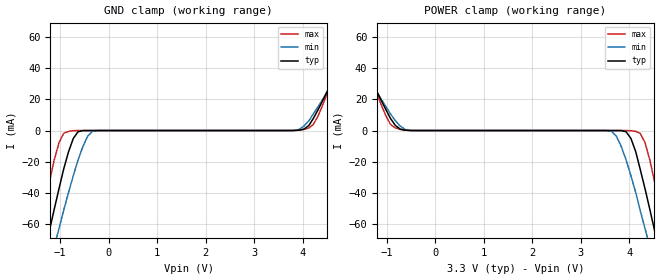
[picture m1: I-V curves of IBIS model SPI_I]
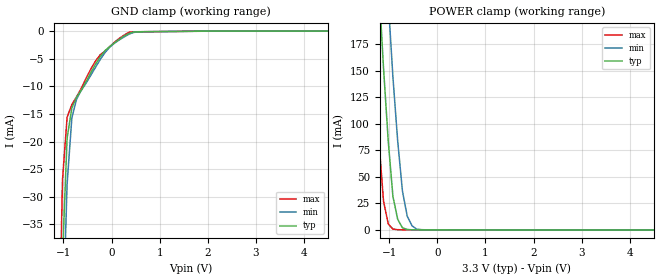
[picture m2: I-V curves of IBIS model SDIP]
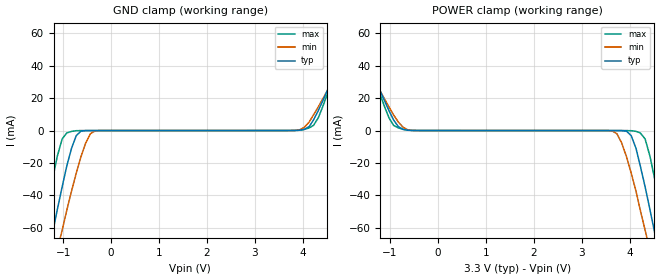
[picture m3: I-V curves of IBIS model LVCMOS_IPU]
|   National Semiconductor Corporation
|   IBIS Model of LMH0387
[IBIS Ver]   4.2
[File name]   lmh0387.ibs
[File Rev]   1.2
[Notes]
 Created By  Pegah Alavi
   Revision History
   1.0  Initial Release
   1.1  Updated SDOP/SDON buffer
   1.2  Updated SPDP and SPIN C_comp values
This model supports the LVCMOS output, LVCMOS Input, SPI input, SPI
output, CML input, and LVDS output on the LMH0387. Static, analog,
and reserved pins are not modeled. Note that the SDIP and SDIN pins
need an external 100ohm termination.
Begin IBIS Parser Results
| Do NOT edit this section manually!
Checking ...\LMH0387.ibs for IBIS 4.2 Compatibility...
WARNING - Combined Pulldown for Model: SDON Typical data is non-monotonic
WARNING - Combined Pulldown for Model: SDON Minimum data is non-monotonic
WARNING - Combined Pulldown for Model: SDON Maximum data is non-monotonic
WARNING - Combined Pulldown for Model: SDOP Typical data is non-monotonic
WARNING - Combined Pulldown for Model: SDOP Minimum data is non-monotonic
WARNING - Combined Pulldown for Model: SDOP Maximum data is non-monotonic
Errors  : 0
Warnings: 6
File Passed
| End IBIS Parser Results
[Date]   09/15/2010
[Source]  Generated by National Semincoductor Corporation.
[Disclaimer]
(C) Copyright National Semiconductor Corporation 2010
   All rights reserved
National Semiconductor Corporation hereby grants the
user of this IBIS model a non-exclusive, nontransferable
license to use this IBIS model under the following terms.
Before using this IBIS model, the user should read this
license.  If the user does not accept these terms,  the
IBIS model should be returned to National within 30 days.
The user is granted this license only to use the
IBIS model and is not granted rights to sell, load, rent,
lease or license the IBIS model in whole or in part, or in
modified form to anyone other than user. User may modify
the IBIS model to suit its specific applications but rights
to derivative works and such modifications shall belong to
National.
This IBIS model is provided on an "AS IS" basis and
National makes absolutely no warranty with respect to the
information contained herein.NATIONAL DISCLAIMS AND CUSTOMER
WAIVES ALL WARRANTIES, EXPRESS OR IMPLIED, INCLUDING
WARRANTIES OF MERCHANTABILITY OR FITNESS FOR A PARTICULAR
PURPOSE. The entire risk as to quality and performance is
with the Customer. ACCORDINGLY, IN NO EVENT SHALL THE
COMPANY BE LIABLE FOR ANY DAMAGES, WHETHER IN CONTRACT OR
TORT,INCLUDING ANY LOST PROFITS OR OTHER INCIDENTAL,
CONSEQUENTIAL, EXEMPLARY, OR PUNITIVE DAMAGES ARISING OUT
OF THE USE OR APPLICATION OF THE IBIS model provided in
this package.Further, National reserves the right to make
changes without notice to any product herein to improve
reliability, function, or design. National does not convey
any license under patent rights or any other intellectual
property rights, including those of third parties.
National is not obligated to provide maintenance or support
for the licensed IBIS model.
[Copyright]  Copyright 2010, National Semiconductor, All Rights Reserved
[Component]  LMH0387
[Manufacturer]  National Semiconductor Corp
[Package]
|   typ   min   max
R_pkg   0   0   0
L_pkg   0   0   0
C_pkg   0   0   0
[Pin]   signal_name   model_name   R_pin   L_pin   C_pin
1   RSVD   NC
2   VCCTX   POWER   1.80e-2   2.969e-10   6.261e-13
3   VCCTX   POWER   1.80e-2   2.969e-10   6.261e-13
4   RSVD   NC
5   RSVD   NC
6   RSVD   NC
7   RSVD   NC
8   BNC_IO   NC   1.60e-2   1.855e-10   3.405e-13
9   RSVD   NC
10   RSVD   NC
11   RSVD   NC
12   RSVD   NC
13   RSVD   NC
14   RSVD   NC
15   RSVD   NC
16   RSVD   NC
17   TERMRX   NC   2.77e-1   1.679e-09   2.691e-13
18   SPI_EN   NC   2.87e-1   1.486e-09   1.329e-13
19   VEE   GND   3.00e-2   2.116e-10   3.185e-12
20   AECP   NC   2.93e-1   1.179e-09   1.128e-13
21   AECN   NC   2.76e-1   1.062e-09   1.103e-13
22   CDB   LVCMOS_O   2.66e-1   1.020e-09   1.143e-13
23   CDTHRESH   NC   2.64e-1   1.004e-09   1.125e-13
24   VEE   GND   3.00e-2   2.116e-10   3.185e-12
25   VEE   GND   3.00e-2   2.116e-10   3.185e-12
26   SSB   LVCMOS_IPU   2.21e-1   7.898e-10   1.088e-13
27   SDOB   SDON   1.22e-1   5.735e-10   1.069e-13
28   SDO   SDOP   1.28e-1   6.293e-10   1.115e-13
29   MISO   SPI_O   2.28e-1   8.392e-10   1.102e-13
30   VCCRX   POWER   1.03e-1   6.790e-10   1.383e-13
31   VEE   GND   3.00e-2   2.116e-10   3.185e-12
32   VEE   GND   3.00e-2   2.116e-10   3.185e-12
33   SDI   SDIP   1.28e-1   7.324e-10   1.327e-13
34   SDIb   SDIN   1.25e-1   7.295e-10   1.360e-13
35   VEE   GND   3.00e-2   2.116e-10   3.185e-12
36   RREF   NC   1.44e-1   8.481e-10   1.239e-13
37   VEE   GND   3.00e-2   2.116e-10   3.185e-12
38   SCK   SPI_I   4.48e-1   2.966e-09   2.892e-13
39   MOSI   SPI_I   4.51e-1   2.840e-09   2.969e-13
40   TX_EN   LVCMOS_IPU   2.25e-1   8.038e-10   1.114e-13
41   VEE   GND   3.00e-2   2.116e-10   3.185e-12
42   RSVD   NC
43   VCCTX   POWER   1.30e-1   9.447e-10   1.625e-13
44   SD_HDb   LVCMOS_IPD   2.72e-1   1.617e-09   1.570e-13
45   TERMTX   NC
46   RSVD   NC
47   RSVD   NC
48   RSVD   NC
[Diff pin]  inv_pin  vdiff  tdelay_typ  tdelay_min  tdelay_max
28   27   0.0   0.0s   0.0s   0.0s
33   34   3.3   0.0s   0.0s   0.0s
| Models and submodels in the file (9): SPI_I (Input), SDIP (Input), SDIN (Input), LVCMOS_IPU (Input), LVCMOS_IPD (Input), SPI_O (Output), LVCMOS_O (Output), SDOP (Output), SDON (Output)
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|   Model SPI_I
[Model]  SPI_I
Model_type Input
Vinl =   0
Vinh =   2
C_comp   542.2fF   513.0fF   577.4fF
[Temperature Range]   25.000   85.000   -40.000
[Voltage Range]   3.300V   3.1350V   3.4650V
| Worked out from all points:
|   GND clamp passes 1 mA (typ) near -0.63 V on its own axis
|   POWER clamp passes 1 mA (typ) near -0.73 V on its own axis
[GND_clamp]
|Voltage   I(typ)   I(min)   I(max)
-3.3V     -364mA     -339mA     -395mA
-1.42V    -92.4mA    -110mA     -65.8mA
-1.22V    -64.4mA    -86.2mA    -33.2mA
-1.02V    -37.2mA    -62.7mA    -7.71mA
-924mV    -24.7mA    -51.1mA    -1.8mA
-627mV    -760uA     -18.8mA    -10.3uA
-330mV    -276nA     -549uA     -1.61nA
4.03V     922uA      2.9mA      717uA
4.32V     13.4mA     15.3mA     9.4mA
5.02V     58.7mA     51.2mA     66.7mA
5.31V     78.6mA     66.8mA     91.9mA
6.6V      165mA      135mA      202mA
[POWER_clamp]
|Voltage   I(typ)   I(min)   I(max)
-3.3V     165mA      135mA      202mA
-2.01V    78.6mA     66.8mA     91.9mA
-1.72V    58.7mA     51.2mA     66.7mA
-1.02V    13.4mA     15.3mA     9.4mA
-726mV    922uA      2.9mA      717uA
3.63V     -276nA     -549uA     -1.61nA
3.93V     -760uA     -18.8mA    -10.3uA
4.13V     -13.7mA    -39.8mA    -535uA
4.32V     -37.2mA    -62.7mA    -7.71mA
4.52V     -64.4mA    -86.2mA    -33.2mA
4.72V     -92.4mA    -110mA     -65.8mA
6.6V      -364mA     -339mA     -395mA
|   Model SDIP
[Model]   SDIP
Model_type   Input
Vinl= 0.8V
Vinh= 2.0V
C_comp   0.5pF   0.5pF   0.5pF
[Temperature Range]   25.0   85.0   -40.0
[Voltage Range]   3.300V   3.135   3.465
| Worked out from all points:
|   POWER clamp passes 1 mA (typ) near -0.66 V on its own axis
[GND Clamp]
|Voltage   I(typ)   I(min)   I(max)
-3.4V     -2.25A     -2.07A     -2.5A
-1.12V    -87.3mA    -103mA     -68.6mA
-1.02V    -41mA      -55.6mA    -27mA
-924mV    -19.4mA    -27.7mA    -15.6mA
-825mV    -13.9mA    -15.7mA    -13.3mA
-726mV    -12mA      -12.3mA    -11.9mA
-429mV    -7.51mA    -7.97mA    -6.84mA
-231mV    -4.59mA    -5.09mA    -4.24mA
-33mV     -2.78mA    -2.86mA    -2.79mA
363mV     -422uA     -559uA     -206uA
1.95V     -14.7uA    -3.4uA     -21.9uA
6.8V      0A         0A         0A
[Power Clamp]
|Voltage   I(typ)   I(min)   I(max)
-3.4V     2.39A      2.36A      2.46A
-1.42V    411mA      540mA      264mA
-1.32V    321mA      455mA      170mA
-1.22V    234mA      372mA      87mA
-1.12V    153mA      291mA      27.4mA
-1.02V    83mA       215mA      5.51mA
-924mV    31.7mA     144mA      864uA
-825mV    10.1mA     84mA       276uA
-726mV    2.05mA     36.7mA     133uA
-627mV    479uA      13.1mA     126uA
-429mV    139uA      763uA      115uA
6.8V      0A         0A         0A
|   Model LVCMOS_IPU
[Model]  LVCMOS_IPU
Model_type Input
Vinl =   0
Vinh =   2
C_comp   542.2fF   513.0fF   577.4fF
[Temperature Range]   25.000   85.000   -40.000
[Voltage Range]   3.300V   3.1350V   3.4650V
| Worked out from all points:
|   GND clamp passes 1 mA (typ) near -0.65 V on its own axis
|   POWER clamp passes 1 mA (typ) near -0.74 V on its own axis
[GND_clamp]
|Voltage   I(typ)   I(min)   I(max)
-3.3V     -377mA     -351mA     -411mA
-1.42V    -92.3mA    -111mA     -63.7mA
-1.22V    -63mA      -86.1mA    -29.9mA
-1.02V    -34.7mA    -61.4mA    -5.21mA
-924mV    -21.9mA    -49.2mA    -1.49mA
-726mV    -3.14mA    -26.2mA    -104uA
-330mV    -14.5uA    -173uA     -20uA
4.03V     720uA      1.99mA     693uA
4.32V     12.2mA     14.5mA     7.75mA
5.02V     60mA       52.7mA     67.4mA
5.21V     73.9mA     63.7mA     85.1mA
6.6V      172mA      142mA      209mA
[POWER_clamp]
|Voltage   I(typ)   I(min)   I(max)
-3.3V     172mA      142mA      209mA
-1.91V    73.9mA     63.7mA     85.1mA
-1.72V    60mA       52.7mA     67.4mA
-1.02V    12.2mA     14.5mA     7.75mA
-726mV    720uA      1.99mA     693uA
3.63V     -14.5uA    -173uA     -20uA
4.03V     -3.14mA    -26.2mA    -104uA
4.22V     -21.9mA    -49.2mA    -1.49mA
4.32V     -34.7mA    -61.4mA    -5.21mA
4.52V     -63mA      -86.1mA    -29.9mA
4.72V     -92.3mA    -111mA     -63.7mA
6.6V      -377mA     -351mA     -411mA
